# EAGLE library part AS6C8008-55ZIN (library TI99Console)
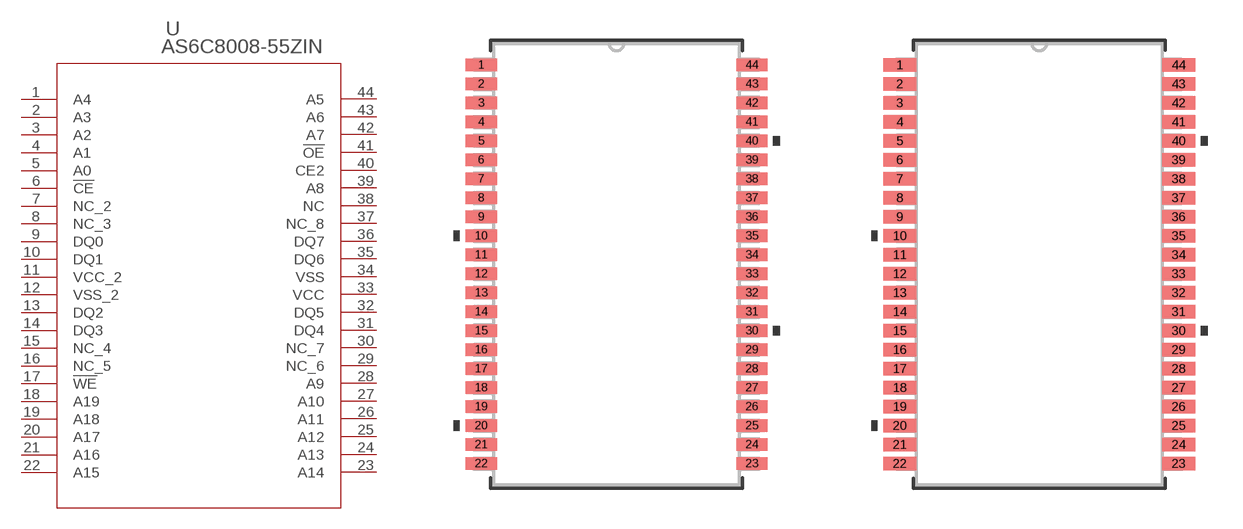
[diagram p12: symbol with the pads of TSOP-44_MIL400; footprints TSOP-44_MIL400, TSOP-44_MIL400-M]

Designator prefix U

## AS6C8008-55ZIN (BUILT_BY: EMA_UL_Team; MANUFACTURER_PART_NUMBER: AS6C8008-55ZIN; VENDOR: Alliance Memory)  [TSOP-44_MIL400]
1  A4  in
2  A3  in
3  A2  in
4  A1  in
5  A0  in
6  !CE  in
7  NC_2  nc
8  NC_3  nc
9  DQ0
10  DQ1
11  VCC_2  pwr
12  VSS_2  pwr
13  DQ2
14  DQ3
15  NC_4  nc
16  NC_5  nc
17  !WE  in
18  A19  in
19  A18  in
20  A17  in
21  A16  in
22  A15  in
23  A14  in
24  A13  in
25  A12  in
26  A11  in
27  A10  in
28  A9  in
29  NC_6  nc
30  NC_7  nc
31  DQ4
32  DQ5
33  VCC  pwr
34  VSS  pwr
35  DQ6
36  DQ7
37  NC_8  nc
38  NC  nc
39  A8  in
40  CE2  in
41  !OE
42  A7  in
43  A6  in
44  A5  in

## AS6C8008-55ZINTSOP-44_MIL400-M (BUILT_BY: EMA_UL_Team; MANUFACTURER_PART_NUMBER: AS6C8008-55ZIN; VENDOR: Alliance Memory)  [TSOP-44_MIL400-M]
Pads as for TSOP-44_MIL400

## AS6C8008-55ZINTSOP-44_MIL400-L (BUILT_BY: EMA_UL_Team; MANUFACTURER_PART_NUMBER: AS6C8008-55ZIN; VENDOR: Alliance Memory)  [TSOP-44_MIL400-L]
Pads as for TSOP-44_MIL400

## Footprint TSOP-44_MIL400 (pad centres in mm)
smd 1.321 x 0.508: 1 -5.702,8.4; 2 -5.702,7.6; 3 -5.702,6.8; 4 -5.702,6; 5 -5.702,5.2; 6 -5.702,4.4; 7 -5.702,3.6; 8 -5.702,2.8; 9 -5.702,2; 10 -5.702,1.2; 11 -5.702,0.4; 12 -5.702,-0.4; 13 -5.702,-1.2; 14 -5.702,-2; 15 -5.702,-2.8; 16 -5.702,-3.6; 17 -5.702,-4.4; 18 -5.702,-5.2; 19 -5.702,-6; 20 -5.702,-6.8; 21 -5.702,-7.6; 22 -5.702,-8.4; 23 5.702,-8.4; 24 5.702,-7.6; 25 5.702,-6.8; 26 5.702,-6; 27 5.702,-5.2; 28 5.702,-4.4; 29 5.702,-3.6; 30 5.702,-2.8; 31 5.702,-2; 32 5.702,-1.2; 33 5.702,-0.4; 34 5.702,0.4; 35 5.702,1.2; 36 5.702,2; 37 5.702,2.8; 38 5.702,3.6; 39 5.702,4.4; 40 5.702,5.2; 41 5.702,6; 42 5.702,6.8; 43 5.702,7.6; 44 5.702,8.4

## Footprint TSOP-44_MIL400-M (pad centres in mm)
smd 1.384 x 0.559: 1 -5.874,8.4; 2 -5.874,7.6; 3 -5.874,6.8; 4 -5.874,6; 5 -5.874,5.2; 6 -5.874,4.4; 7 -5.874,3.6; 8 -5.874,2.8; 9 -5.874,2; 10 -5.874,1.2; 11 -5.874,0.4; 12 -5.874,-0.4; 13 -5.874,-1.2; 14 -5.874,-2; 15 -5.874,-2.8; 16 -5.874,-3.6; 17 -5.874,-4.4; 18 -5.874,-5.2; 19 -5.874,-6; 20 -5.874,-6.8; 21 -5.874,-7.6; 22 -5.874,-8.4; 23 5.874,-8.4; 24 5.874,-7.6; 25 5.874,-6.8; 26 5.874,-6; 27 5.874,-5.2; 28 5.874,-4.4; 29 5.874,-3.6; 30 5.874,-2.8; 31 5.874,-2; 32 5.874,-1.2; 33 5.874,-0.4; 34 5.874,0.4; 35 5.874,1.2; 36 5.874,2; 37 5.874,2.8; 38 5.874,3.6; 39 5.874,4.4; 40 5.874,5.2; 41 5.874,6; 42 5.874,6.8; 43 5.874,7.6; 44 5.874,8.4

## Footprint TSOP-44_MIL400-L (pad centres in mm)
smd 0.978 x 0.457: 1 -5.671,8.4; 2 -5.671,7.6; 3 -5.671,6.8; 4 -5.671,6; 5 -5.671,5.2; 6 -5.671,4.4; 7 -5.671,3.6; 8 -5.671,2.8; 9 -5.671,2; 10 -5.671,1.2; 11 -5.671,0.4; 12 -5.671,-0.4; 13 -5.671,-1.2; 14 -5.671,-2; 15 -5.671,-2.8; 16 -5.671,-3.6; 17 -5.671,-4.4; 18 -5.671,-5.2; 19 -5.671,-6; 20 -5.671,-6.8; 21 -5.671,-7.6; 22 -5.671,-8.4; 23 5.671,-8.4; 24 5.671,-7.6; 25 5.671,-6.8; 26 5.671,-6; 27 5.671,-5.2; 28 5.671,-4.4; 29 5.671,-3.6; 30 5.671,-2.8; 31 5.671,-2; 32 5.671,-1.2; 33 5.671,-0.4; 34 5.671,0.4; 35 5.671,1.2; 36 5.671,2; 37 5.671,2.8; 38 5.671,3.6; 39 5.671,4.4; 40 5.671,5.2; 41 5.671,6; 42 5.671,6.8; 43 5.671,7.6; 44 5.671,8.4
